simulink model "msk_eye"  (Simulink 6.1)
settings: Solver=ode45  StartTime=0.0  StopTime=10.0  RelTol=1e-3
libraries: commchan2 x1, commrandsrc2 x1, commsink2 x1, commdigbbndcpm2 x1

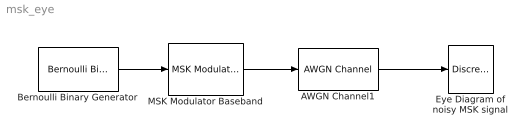
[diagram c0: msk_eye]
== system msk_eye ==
  AWGN Channel1 : commchan2/AWGN Channel  seed=1237  noiseMode="Signal to noise ratio  (SNR)"  EbNodB=10  EsNodB=10  SNRdB=30  bitsPerSym=1  Ps=1  Tsym=1  variance=1
  Bernoulli Binary Generator : commrandsrc2/Bernoulli Binary Generator  P=0.5  seed=61  Ts=0.5  frameBased=off  sampPerFrame=1  orient=off
  Eye Diagram of noisy MSK signal : commsink2/Discrete-Time Eye Diagram Scope  Tag=EyeDiagram  sampPerSymb=8  offsetEye=4  symbPerTrace=4  numTraces=40  numNewFrames=10  LineStyles=-  LineColors=m  dupPoints=on  fading=on  render=on  AxisGrid=on  yMin=-1.5  yMax=1.5  inphaseLabel=In-phase Amplitude  quadratureLabel=Quadrature Amplitude  openScopeAtSimStart=on  dispDiagram=In-phase and Quadrature  FrameNumber=off  FigPos=[512 225 358 412]  figTitle=Eye Diagram  block_type_=eye  numLinesMax=8
  MSK Modulator Baseband : commdigbbndcpm2/MSK Modulator Baseband  inputType=Bit  phaseOffset=0  samplesPerSymbol=8
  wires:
  Bernoulli Binary Generator/1 -> MSK Modulator Baseband/1
  MSK Modulator Baseband/1 -> AWGN Channel1/1
  AWGN Channel1/1 -> Eye Diagram of noisy MSK signal/1
